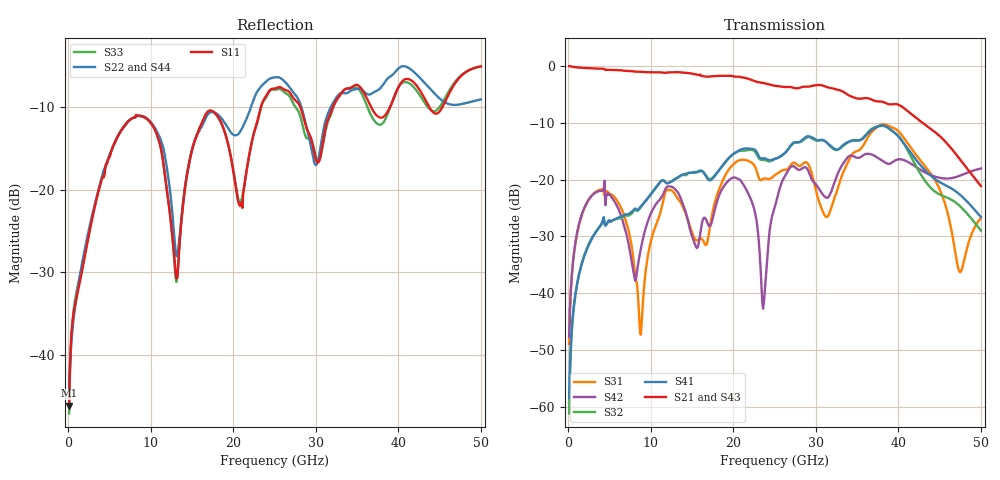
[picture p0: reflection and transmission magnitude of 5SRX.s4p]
! DAC39RF10ACK
! 256-pin FCBGA package
! Texas Instruments 8/20/2022
! Single-ended  S-parameters
! PORT#  PORT_NAME  NET_NAME
! PORT1:  xSRXN.DIEBUMP  xSRXN
! PORT2:  xSRXN.BGA  xSRXN
! PORT3:  xSRXP.DIEBUMP  xSRXP
! PORT4:  xSRXP.BGA  xSRXP
! Touchstone Ver. 1.0
! Number of ports is 4
# Hz	S	MA	R	50.000000
! SCATTERING PARAMETERS  :
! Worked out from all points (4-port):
!   500 points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, 100 MHz to 50 GHz, reference 50 ohm
!   strongest paths, dB at 100 MHz, 12.6 GHz, 25.1 GHz, 37.6 GHz, 50 GHz:
!     S21: 0.0, -1.1, -3.5, -6.2, -21.1
!     S43: 0.0, -1.1, -3.5, -6.1, -21.4
!     S41: -58.5, -20.3, -16.3, -10.6, -26.6
!     S32: -61.2, -20.2, -16.3, -10.6, -29.0
!     S42: -47.8, -21.3, -24.5, -16.3, -18.1
!     S31: -49.0, -22.0, -19.2, -10.6, -26.8
!   lowest |S11| = -46.2 dB at 100 MHz (marker M1), VSWR 1.01, Z = 50.4 + j0.289 ohm
!   |S11| at or under -10 dB: start of sweep to 23.33 GHz; 28.12 GHz to 32.05 GHz (3.929 GHz wide, 13.1 % of centre); 36.71 GHz to 38.98 GHz (2.265 GHz wide, 5.99 % of centre)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
1e8  0.004921 35.6  0.9883 -2.8  0.003364 84.8  0.0009664 -96.6
     0.9955 -2.6  0.006065 27.2  0.001137 -99.5  0.004154 80.6
     0.003563 83.9  0.0008732 -100.4  0.004418 32.7  0.9935 -2.8
     0.001187 -99.4  0.004094 73.0  0.996 -2.5  0.005488 34.5
3e9  0.07076 29.3  0.9487 -68.9  0.07478 16.6  0.03142 -170.6
     0.9511 -68.7  0.07397 -11.0  0.03173 -170.0  0.07395 20.1
     0.07435 16.8  0.03178 -170.5  0.0718 28.9  0.9486 -68.9
     0.03138 -170.2  0.07389 20.1  0.9509 -68.7  0.07501 -10.3
7.8e9  0.2717 -74.1  0.8945 -176.0  0.02271 -99.0  0.05172 85.5
       0.8971 -175.9  0.272 -100.2  0.05226 85.2  0.01647 -132.6
       0.02249 -99.4  0.05121 85.7  0.2726 -74.0  0.8948 -176.0
       0.05283 85.1  0.0168 -134.5  0.9 -175.9  0.2718 -100.2
1.56e10  0.2152 -78.7  0.8355 9.5  0.02813 167.3  0.1179 -90.7
         0.8384 9.4  0.2147 -87.2  0.1157 -90.7  0.02473 30.0
         0.02907 167.0  0.1165 -90.2  0.2173 -80.7  0.8371 9.4
         0.1162 -91.1  0.02495 29.2  0.8399 9.3  0.2147 -85.3
2.35e10  0.3357 -50.0  0.7128 -169.0  0.1007 -144.5  0.1533 83.9
         0.7104 -168.7  0.4303 -115.9  0.1483 85.0  0.00921 -141.0
         0.09994 -143.7  0.1489 84.7  0.3324 -49.8  0.7103 -168.9
         0.1528 84.1  0.008593 -144.7  0.7122 -169.0  0.4321 -115.2
3.13e10  0.2521 -83.3  0.652 16.2  0.04631 -140.3  0.2135 -102.4
         0.6517 16.7  0.2744 -114.3  0.2126 -101.5  0.06989 -157.0
         0.04671 -139.1  0.2129 -101.8  0.242 -81.4  0.6513 17.5
         0.2118 -102.3  0.06903 -157.2  0.6454 18.0  0.2721 -117.2
5e10  0.5605 -125.1  0.07808 -13.8  0.04344 134.4  0.03483 -152.6
      0.0877 -14.5  0.3531 -160.4  0.04954 -172.1  0.1247 56.8
      0.04575 133.3  0.03553 -158.2  0.5581 -123.8  0.07682 -14.3
      0.04679 -167.7  0.125 55.6  0.08527 -14.2  0.3532 -161.8
